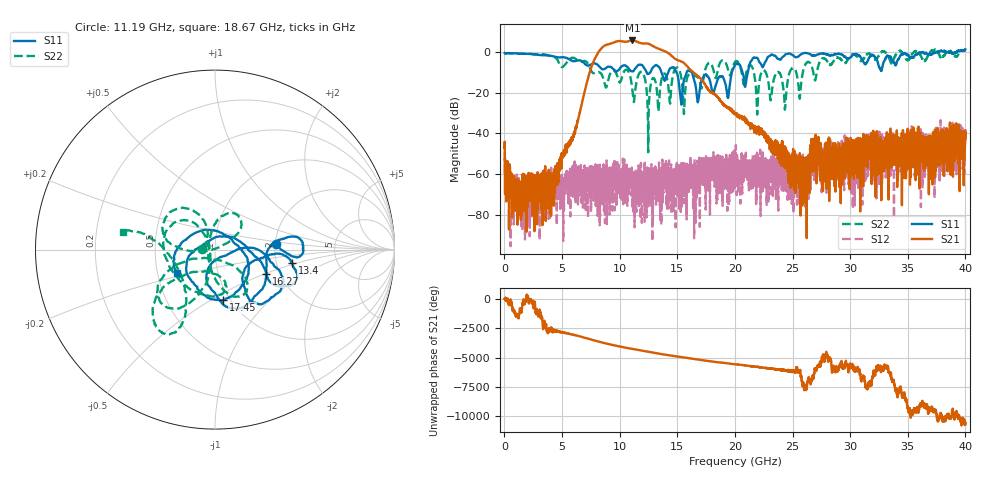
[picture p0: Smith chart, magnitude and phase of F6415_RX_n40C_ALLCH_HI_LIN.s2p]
!Keysight Technologies,N5245B,MY52451815,A.15.70.20
!Date: Wednesday, April 17, 2024 15:39:08
!Correction: S33(C  2-Port  )
!S43(C  2-Port  )
!S34(C  2-Port  )
!S44(C  2-Port  )
!S2P File: Measurements: S33, S43, S34, S44:
# Hz S  RI  R 50
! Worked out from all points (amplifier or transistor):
!   4000 points, 10 MHz to 40 GHz, reference 50 ohm
!   highest |S21| = 5.8 dB at 11.1 GHz (marker M1)
!   |S21| within 3 dB of that: 8.572 GHz to 12.96 GHz (4.391 GHz wide, 40.8 % of centre)
!   unconditionally stable (mu >= 1): start of sweep to 32.7 GHz; 33.06 GHz to 34.07 GHz; 34.47 GHz to 35.52 GHz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
!   at 6.67 GHz: K = 5944.97, MAG = -22.4 dB, |S12| = -63.0 dB
!   at 20.01 GHz: K = 12567.42, MAG = -27.2 dB, |S12| = -63.7 dB
!   at 40 GHz: K = 239.07, MSG = -1.0 dB, |S12| = -37.8 dB
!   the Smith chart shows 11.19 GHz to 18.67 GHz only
!   S11 on the Smith chart (normalised r, x): 11.19 GHz: 2.02, +0.15; 13.4 GHz: 2.44, -0.45; 16.27 GHz: 1.70, -0.51; 17.45 GHz: 0.93, -0.57; 18.67 GHz: 0.63, -0.18
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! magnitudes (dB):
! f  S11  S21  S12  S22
! 10 MHz  -0.4  -47.1  -49.3  -0.6
! 650 MHz  -0.5  -71.5  -70.9  -0.7
! 4.08 GHz  -1.8  -63.1  -61.7  -2.1
! 6.68 GHz  -4.3  -26.1  -70.5  -4.7
! 8.3 GHz  -7.4  1.2  -64.6  -10.1
! 11.1 GHz  -9.5  5.8  -68.4  -18.5
! 11.19 GHz  -9.3  5.7  -61.4  -23.1
! 11.87 GHz  -6.2  4.3  -63.9  -9.7
! 13.34 GHz  -7.0  1.8  -59.2  -28.2
! 13.4 GHz  -7.2  1.7  -59.9  -25.8
! 15.32 GHz  -23.9  -4.5  -60.1  -11.7
! 16.27 GHz  -10.0  -9.3  -57.6  -11.3
! 16.78 GHz  -24.7  -11.7  -64.1  -12.3
! 17.45 GHz  -10.9  -16.4  -52.7  -8.0
! 18.67 GHz  -12.1  -23.3  -59.9  -5.6
! 19.4 GHz  -22.5  -27.4  -61.7  -8.7
! 20.01 GHz  -6.3  -30.1  -63.7  -4.8
! 24.34 GHz  -1.4  -57.2  -63.0  -28.0
! 26.03 GHz  -0.4  -58.8  -56.8  -6.9
! 26.67 GHz  -1.5  -51.2  -60.3  -7.1
! 33.34 GHz  -2.2  -52.0  -51.0  -2.5
! 40 GHz  1.4  -39.9  -37.8  0.7
